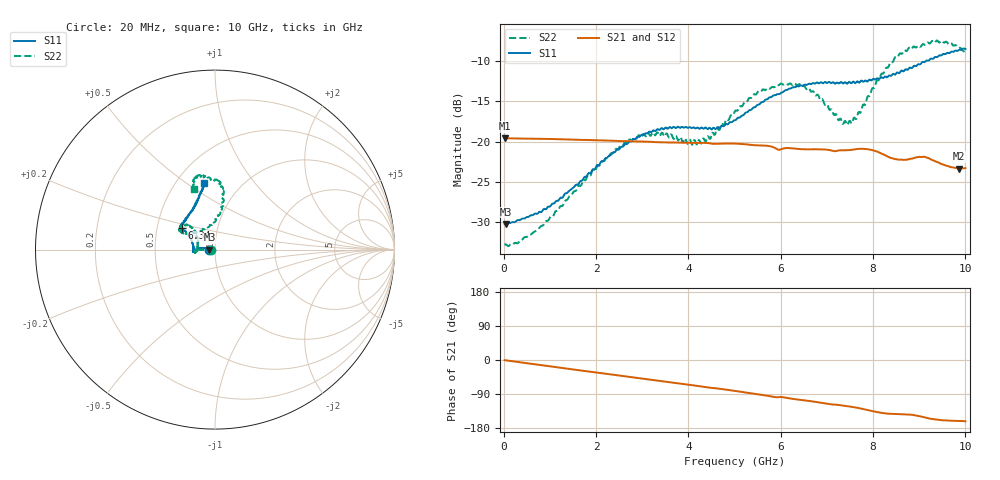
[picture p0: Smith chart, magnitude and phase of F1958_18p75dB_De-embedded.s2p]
! Integrated Device Technology
! Corporate Headquarters
! 6024 Silver Creek Valley Road
! San Jose, CA 95138  USA
! Phone:  1-408-284-8200
! Toll Free:  1-800-223-1366
! Webpage:  http://www.idt.com/
! Timing and RF Division
! 515 Groton Road, Suite 102
! Westford, MA 01886-6024
! Device:  F1958
! Description: 7-bit 0.25 dB Digital Step Attenuator
! Frequency:  0.001 -  6.000 GHz
! Package:  4x4 mm Thin QFN Plastic Package: 24 pin
! Ports:  2 RF, 12 DC
!  Pin  1  = D0
!  Pin  2  = VDD
!  Pin  3  = VMODE
!  Pin  4  = GND
!  Pin  5  = RF1  =  Port 1
!  Pin  6  = GND
!  Pin  7  = GND
!  Pin  8  = GND
!  Pin  9  = GND
!  Pin 10  = GND
!  Pin 11  = GND
!  Pin 12  = GND
!  Pin 13  = GND
!  Pin 14  = RF2  =  Port 2
!  Pin 15  = GND
!  Pin 16  = LE
!  Pin 17  = CLK
!  Pin 18  = DATA
!  Pin 19  = D6
!  Pin 20  = D5
!  Pin 21  = D4
!  Pin 22  = D3
!  Pin 23  = D2
!  Pin 24  = D1
! State:  75
! Atten State:  18.75 dB
! Voltage:  +3.30 Volts
! Current:  0.258 mA
! Data:  The device was measured on a F1958 evaluation board which has
!  individual transmission lines to the RF pins.  Data was collected
!  using a calibrated network analyzer.  The evaluation board was
!  de-embedded using Automatic Fixture Removal (AFR).
!  The reference plane is the edge of the package pin.
! Misc:
!  Action Tracker AT0419
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# GHz S dB R 50
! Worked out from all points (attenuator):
!   500 points, 20 MHz to 10 GHz, reference 50 ohm
!   highest |S21| = -19.57 dB at 20 MHz (marker M1); lowest = -23.3 dB at 9.86 GHz (marker M2)
!   lowest |S11| = -30.2 dB at 40 MHz (marker M3), VSWR 1.06, Z = 47 - j0.0429 ohm
!   |S11| at or under -10 dB: start of sweep to 9.141 GHz
!   |S22| runs from -33.0 to -7.4 dB; largest |S21 - S12| = 0.00043
!   S11 on the Smith chart (normalised r, x): 20 MHz: 0.94, -0.00; 6.34 GHz: 0.67, +0.17; 10 GHz: 0.68, +0.59
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0.02  -30.18 -178.9  -19.57 -0.4  -19.57 -0.4  -32.82 -178.1
0.04  -30.22 -179.2  -19.57 -0.8  -19.57 -0.7  -32.75 -177.2
0.32  -29.74 175.3  -19.61 -5.4  -19.60 -5.4  -32.53 179.3
0.72  -28.97 173.0  -19.64 -12.0  -19.63 -12.0  -30.96 -179.5
1.7  -24.84 171.6  -19.78 -28.0  -19.77 -28.0  -25.09 179.3
2.6  -20.53 177.4  -19.93 -42.6  -19.91 -42.6  -20.30 -177.4
2.92  -19.39 -178.9  -19.97 -47.8  -19.95 -47.9  -19.21 -174.5
3.36  -18.52 -175.4  -20.07 -55.0  -20.07 -55.1  -19.14 -170.8
4.24  -18.41 -179.0  -20.15 -69.0  -20.16 -69.1  -19.83 166.4
4.64  -18.17 171.9  -20.26 -75.3  -20.27 -75.4  -18.38 148.3
5.02  -17.33 160.8  -20.24 -81.8  -20.25 -81.8  -16.12 137.7
5.56  -15.23 150.4  -20.46 -91.2  -20.47 -91.3  -13.83 138.4
6.34  -13.14 147.5  -20.88 -104.0  -20.90 -103.9  -12.99 151.6
6.68  -12.77 146.3  -20.95 -109.2  -20.96 -109.1  -13.77 151.6
7.3  -12.59 140.5  -21.07 -119.5  -21.08 -119.3  -17.14 129.5
7.48  -12.57 137.4  -21.04 -122.5  -21.04 -122.4  -17.45 111.0
7.68  -12.58 134.9  -20.90 -126.6  -20.89 -126.5  -16.36 94.2
8.34  -11.79 118.8  -21.90 -141.8  -21.91 -141.9  -10.65 80.4
8.68  -11.15 112.1  -22.25 -143.4  -22.26 -143.3  -8.62 85.2
9.26  -9.67 104.4  -22.23 -155.4  -22.23 -155.4  -7.60 98.5
9.86  -8.61 99.5  -23.33 -160.8  -23.35 -160.7  -8.36 107.9
10  -8.48 99.5  -23.28 -161.8  -23.30 -161.5  -8.91 108.8
